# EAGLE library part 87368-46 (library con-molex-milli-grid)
RECEPTACAL
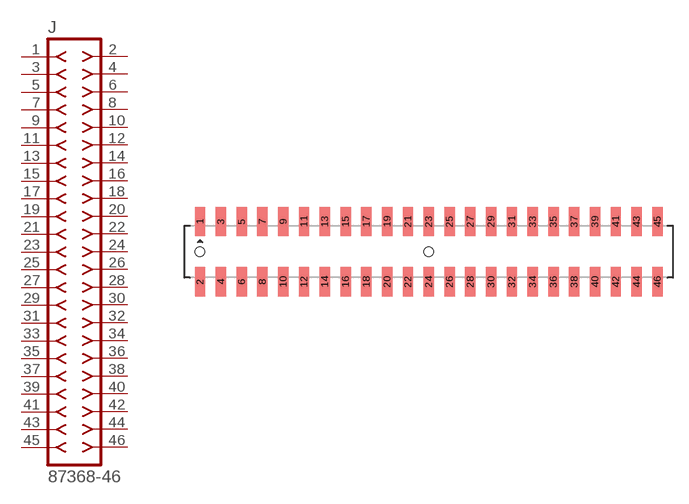
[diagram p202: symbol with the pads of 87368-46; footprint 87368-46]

Designator prefix J

## 87368-46  [87368-46]
1  1  pas
2  2  pas
3  3  pas
4  4  pas
5  5  pas
6  6  pas
7  7  pas
8  8  pas
9  9  pas
10  10  pas
11  11  pas
12  12  pas
13  13  pas
14  14  pas
15  15  pas
16  16  pas
17  17  pas
18  18  pas
19  19  pas
20  20  pas
21  21  pas
22  22  pas
23  23  pas
24  24  pas
25  25  pas
26  26  pas
27  27  pas
28  28  pas
29  29  pas
30  30  pas
31  31  pas
32  32  pas
33  33  pas
34  34  pas
35  35  pas
36  36  pas
37  37  pas
38  38  pas
39  39  pas
40  40  pas
41  41  pas
42  42  pas
43  43  pas
44  44  pas
45  45  pas
46  46  pas

## Footprint 87368-46 (pad centres in mm)
RECEPTACAL SMD Dual Row, Side Entry
smd 1 x 2.8: 1 -22,2.9; 2 -22,-2.9; 3 -20,2.9; 4 -20,-2.9; 5 -18,2.9; 6 -18,-2.9; 7 -16,2.9; 8 -16,-2.9; 9 -14,2.9; 10 -14,-2.9; 11 -12,2.9; 12 -12,-2.9; 13 -10,2.9; 14 -10,-2.9; 15 -8,2.9; 16 -8,-2.9; 17 -6,2.9; 18 -6,-2.9; 19 -4,2.9; 20 -4,-2.9; 21 -2,2.9; 22 -2,-2.9; 23 0,2.9; 24 0,-2.9; 25 2,2.9; 26 2,-2.9; 27 4,2.9; 28 4,-2.9; 29 6,2.9; 30 6,-2.9; 31 8,2.9; 32 8,-2.9; 33 10,2.9; 34 10,-2.9; 35 12,2.9; 36 12,-2.9; 37 14,2.9; 38 14,-2.9; 39 16,2.9; 40 16,-2.9; 41 18,2.9; 42 18,-2.9; 43 20,2.9; 44 20,-2.9; 45 22,2.9; 46 22,-2.9
hole 0.914 at -22,0
hole 0.914 at 0,0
